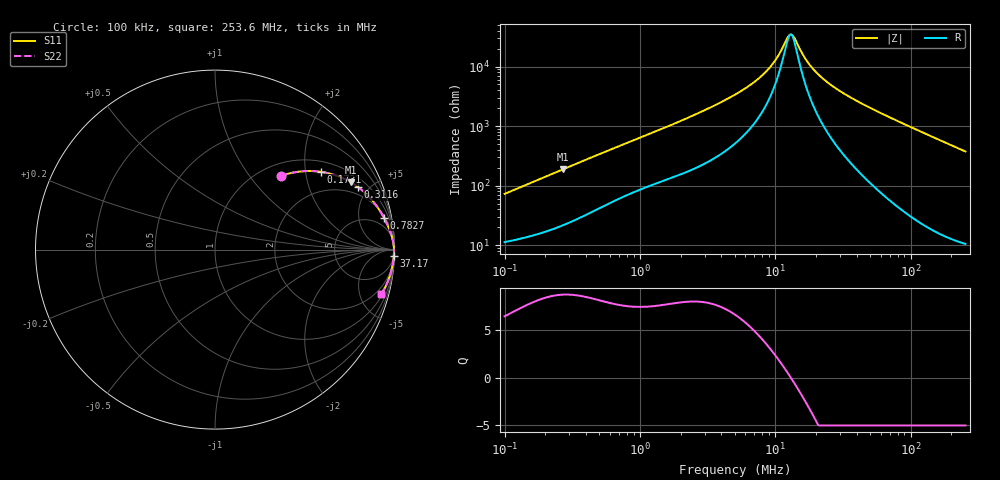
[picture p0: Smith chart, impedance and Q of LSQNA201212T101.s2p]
! LSQNA201212T101  S-PARAMETER MODEL  ( General Type )
! Model Generated by TAIYO YUDEN Corporation (http://www.ty-top.com)
! Version 2.0
! TAIYO YUDEN Control No. 100810NF25SB-FKC
! Copyright(c) 2007 TAIYO YUDEN CO.,LTD. All Rights Reserved.
! Product Description (link to TY-COMPAS)
! https://ds.yuden.co.jp/TYCOMPAS/or/detail?pn=LSQNA201212T101K&u=M
! Products Name : Inductors
! Characteristics :
!  Inductance : 100 uH , SRF(min) : 8.0 MHz , DC Resistance(max) : 9.1 Ohm
!  Rated Current : Saturation :60 mA , Temp Rise : 130 mA (40 degC)
!  Case Size : 2.0 x 1.25 / 0.079 x 0.049 [mm/inch] , Thickness : 1.25 / 0.049 [mm/inch]
!  (Conditions: Temperature = 25 degC , DC Bias Current/Voltage = 0A / 0V)
! External Node Assignments :
!  1  o---GGG---o  2
! GND o---------o GND
! Frequency Range : 0.1MHz  -  253.640152MHz  [ 402 STEP ]
# MHz S RI R 50
! Freq[MHz].  S11 Real  S11 Imag  S21 Real  S21 Imag  S12 Real  S12 Imag  S22 Real  S22 Imag
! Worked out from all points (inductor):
!   401 points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, 100 kHz to 253.6 MHz, reference 50 ohm
!   read as one part in series: L = 113 uH near 104 kHz
!   highest Q = 8.65 at 271.7 kHz (marker M1), where L = 110 uH
!   self-resonance near 12.9 MHz
!   S11 on the Smith chart (normalised r, x): 100 kHz: 1.23, +1.44; 173.1 kHz: 1.30, +2.44; 311.6 kHz: 1.50, +4.29; 782.7 kHz: 2, +10; 37.17 MHz: 5, -58; 253.6 MHz: 1.21, -7.49
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0.1  0.3657 0.4097  0.6343 -0.4097  0.6343 -0.4097  0.3657 0.4097
0.173099  0.5901 0.4334  0.4099 -0.4334  0.4099 -0.4334  0.5901 0.4334
0.271668  0.7573 0.3748  0.2427 -0.3748  0.2427 -0.3748  0.7573 0.3748
0.31161  0.7971 0.3484  0.2029 -0.3484  0.2029 -0.3484  0.7971 0.3484
0.371712  0.8399 0.3125  0.1601 -0.3125  0.1601 -0.3125  0.8399 0.3125
0.782721  0.9407 0.1785  0.0593 -0.1785  0.0593 -0.1785  0.9407 0.1785
1.381698  0.9722 0.1108  0.0278 -0.1108  0.0278 -0.1108  0.9722 0.1108
2.909469  0.99 0.0546  0.01 -0.0546  0.01 -0.0546  0.99 0.0546
5.03627  0.9947 0.029  0.0053 -0.029  0.0053 -0.029  0.9947 0.029
6.890928  0.996 0.0181  0.004 -0.0181  0.004 -0.0181  0.996 0.0181
8.717747  0.9966 0.011  0.00341 -0.011  0.00341 -0.011  0.9966 0.011
10.19738  0.9969 0.00662  0.00314 -0.00662  0.00314 -0.00662  0.9969 0.00662
12.1642  0.9971 0.0018  0.00293 -0.0018  0.00293 -0.0018  0.9971 0.0018
12.90076  0.9971 0.000205  0.00288 -0.000205  0.00288 -0.000205  0.9971 0.000205
13.68191  0.9972 -0.00139  0.00285 0.00139  0.00285 0.00139  0.9972 -0.00139
16.32081  0.9972 -0.00624  0.00279 0.00624  0.00279 0.00624  0.9972 -0.00624
18.72042  0.9972 -0.0101  0.0028 0.0101  0.0028 0.0101  0.9972 -0.0101
24.62993  0.997 -0.0186  0.00298 0.0186  0.00298 0.0186  0.997 -0.0186
37.16932  0.9962 -0.0342  0.0038 0.0342  0.0038 0.0342  0.9962 -0.0342
69.58603  0.9922 -0.0701  0.00781 0.0701  0.00781 0.0701  0.9922 -0.0701
135.4817  0.9767 -0.1378  0.0233 0.1378  0.0233 0.1378  0.9767 -0.1378
253.6402  0.9275 -0.2457  0.0725 0.2457  0.0725 0.2457  0.9275 -0.2457
